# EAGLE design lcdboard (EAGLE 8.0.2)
two capacitors for regulator (in & out) 10uF each
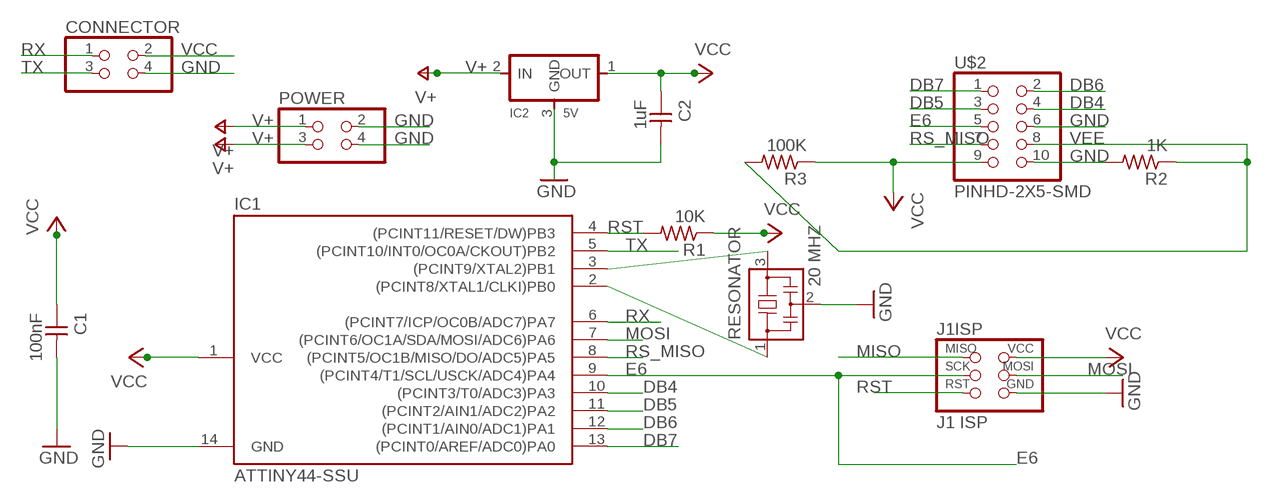
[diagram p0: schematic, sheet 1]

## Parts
C1  100nF  CAP-UNPOLARIZEDFAB  [C1206FAB]
C2  1uF  CAP-UNPOLARIZEDFAB  [C1206FAB]
CONNECTOR  PINHD-2X2-SMD  [2X02SMD]
IC1  ATTINY44-SSU  [SOIC14]
IC2  5V  REGULATORSOT23  [SOT23]
J1ISP  J1 ISP  AVRISPSMD  [2X03SMD]
POWER  PINHD-2X2-SMD  [2X02SMD]
R1  10K  RES-US1206FAB  [R1206FAB]
R2  1K  RES-US1206FAB  [R1206FAB]
R3  100K  RES-US1206FAB  [R1206FAB]
RESONATOR  20 MHZ  RESONATOR  [EFOBM]
U$2  PINHD-2X5-SMD  [2X05SMD]

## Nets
DB4: IC1.10((PCINT3/T0/ADC3)PA3) U$2.4
DB5: IC1.11((PCINT2/AIN1/ADC2)PA2) U$2.3
DB6: IC1.12((PCINT1/AIN0/ADC1)PA1) U$2.2
DB7: IC1.13((PCINT0/AREF/ADC0)PA0) U$2.1
E6: IC1.9((PCINT4/T1/SCL/USCK/ADC4)PA4) J1ISP.3(SCK) U$2.5
GND: C1.2 C2.2 CONNECTOR.4 IC1.14(GND) IC2.3(GND) J1ISP.6(GND) POWER.2 POWER.4 R2.2 RESONATOR.2 U$2.6 U$2.10
MISO: J1ISP.1(MISO)
MOSI: IC1.7((PCINT6/OC1A/SDA/MOSI/ADC6)PA6) J1ISP.4(MOSI)
N$2: IC1.2((PCINT8/XTAL1/CLKI)PB0) RESONATOR.1
N$3: IC1.3((PCINT9/XTAL2)PB1) RESONATOR.3
RS_MISO: IC1.8((PCINT5/OC1B/MISO/DO/ADC5)PA5) U$2.7
RST: IC1.4((PCINT11/RESET/DW)PB3) J1ISP.5(RST) R1.2
RX: CONNECTOR.1 IC1.6((PCINT7/ICP/OC0B/ADC7)PA7)
TX: CONNECTOR.3 IC1.5((PCINT10/INT0/OC0A/CKOUT)PB2)
V+: IC2.2(IN) POWER.1 POWER.3
VCC: C1.1 C2.1 CONNECTOR.2 IC1.1(VCC) IC2.1(OUT) J1ISP.2(VCC) R1.1 R3.1 U$2.9
VEE: R2.1 R3.2 U$2.8

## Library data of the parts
C1 C2 = fab:CAP-UNPOLARIZED
CONNECTOR POWER = fab:PINHD-2X2-SMD
IC1 = fab:ATTINY44
IC2 = fab:REGULATOR
J1ISP = fab:AVRISP
R1-R3 = fab:RES-US: Resistor (US Symbol)
RESONATOR = fab:RESONATOR
U$2 = fab:PINHD-2X5-SMD

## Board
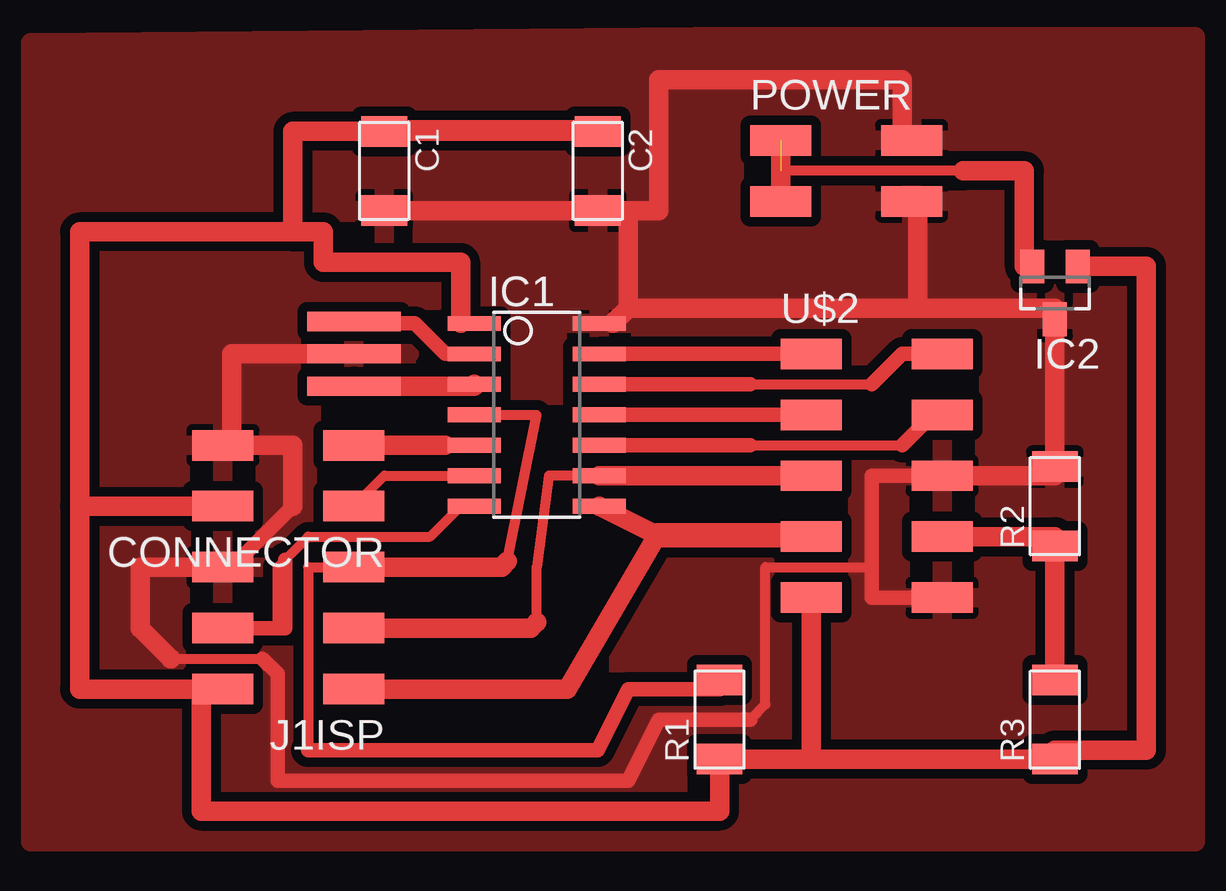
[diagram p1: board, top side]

No outline drawn. Coordinates in mm, seen from the top.
Copper layers (1*16): Top 0.035mm / dielectric 1.5mm / Bottom 0.035mm
Design rules "default *": minimum track width 16mil, minimum drill 24mil, track to track 16mil, track to pad 16mil, pad to pad 16mil, via to via 16mil, smd to smd 8mil, copper to edge 40mil, drill to drill 8mil, minimum pad ring 10mil, minimum via ring 8mil, stop-mask expansion 4mil, vias tented up to drill 0mil, thermal gap 10mil

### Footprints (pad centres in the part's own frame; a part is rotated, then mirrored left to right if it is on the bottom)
C1206FAB = smd 1.27 x 1.905: 1 -1.651,0; 2 1.651,0
2X02SMD = smd 2.54 x 1.27: 1 -2.54,1.27; 2 2.92,1.27; 3 -2.54,-1.27; 4 2.92,-1.27
SOIC14 = smd 0.61 x 2.21: 1 -3.81,-2.603; 2 -2.54,-2.603; 3 -1.27,-2.603; 4 0,-2.603; 5 1.27,-2.603; 6 2.54,-2.603; 7 3.81,-2.603; 8 3.81,2.603; 9 2.54,2.603; 10 1.27,2.603; 11 0,2.603; 12 -1.27,2.603; 13 -2.54,2.603; 14 -3.81,2.603
SOT23 = smd 1 x 1.4: 1 -0.95,-1.1; 2 0.95,-1.1; 3 0,1.1
2X03SMD = smd 2.54 x 1.27: 1 -2.54,2.54; 2 2.92,2.54; 3 -2.54,0; 4 2.92,0; 5 -2.54,-2.54; 6 2.92,-2.54
R1206FAB = smd 1.27 x 1.905: 1 -1.651,0; 2 1.651,0
EFOBM = smd 0.8 x 3.9: 1 -1.35,0; 2 0,0; 3 1.35,0
2X05SMD = smd 2.54 x 1.27: 1 -2.54,2.54; 2 2.92,2.54; 3 -2.54,0; 4 2.92,0; 5 -2.54,-2.54; 6 2.92,-2.54; 7 -2.54,-5.08; 8 2.92,-5.08; 9 -2.54,-7.62; 10 2.92,-7.62

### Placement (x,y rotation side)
C1  13.97,30.48 270 top
C2  22.86,30.48 270 top
CONNECTOR  10.16,17.78 180 top
IC1  20.32,20.32 270 top
IC2  41.91,25.4 180 top
J1ISP  10.16,11.43 180 top
POWER  33.02,30.48 0 top
R1  27.94,7.62 90 top
R2  41.91,16.51 90 top
R3  41.91,7.62 90 top
RESONATOR  12.7,22.86 270 top
U$2  34.29,20.32 0 top

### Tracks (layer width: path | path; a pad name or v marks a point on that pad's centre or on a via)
DB4
  Top 0.406: 29.21,19.05 35.56,19.05 | 36.83,20.32 U$2.4
  Top 0.61: 36.83,20.32 35.56,19.05 | IC1.10 29.21,19.05
DB5
  Top 0.61: U$2.3 IC1.11
DB6
  Top 0.406: U$2.2 36.83,22.86 | 29.21,21.59 34.29,21.59
  Top 0.61: IC1.12 29.21,21.59 | 34.29,21.59 35.56,22.86 U$2.2
DB7
  Top 0.61: U$2.1 IC1.13
E6
  Top 0.406: IC1.9 20.83,17.78 20.32,13.97 20.32,11.68 20.32,11.43 J1ISP.3
  Top 0.813: U$2.5 IC1.9 | J1ISP.3 20.07,11.43 20.32,11.68
GND
  Top 0.406: 13.97,28.57 C1.2 | 35.56,33.02 35.56,31.75 POWER.2 | 10.79,22.86 RESONATOR.2 | 34.92,17.78 U$2.6 | 36.83,12.7 U$2.10 | 36.2,29.21 POWER.4 | 41.91,24.77 IC2.3 R2.2 41.91,17.78 | 9.53,9.53 9.53,6.35 | 29.21,7.62 29.84,8.26 29.84,13.97 34.29,13.97 | 6.99,13.97 J1ISP.6 7.62,13.97 | 5.08,10.16 8.89,10.16
  Top 0.61: U$2.6 34.29,17.78 34.29,13.97 34.29,12.7 38.1,12.7 | 29.21,7.62 25.4,7.62 24.13,5.08 9.53,5.08 9.53,9.53 8.89,10.16 | 10.16,16.51 7.62,13.97
  Top 0.813: 36.2,24.77 36.2,29.21 | 41.91,24.77 36.2,24.77 | 24.13,24.77 23.5,24.13 | 36.2,24.77 24.13,24.77 | IC2.3 41.91,17.78 U$2.6 | C2.2 25.4,28.83 25.4,34.29 35.56,34.29 35.56,31.75 | 10.79,22.86 7.62,22.86 7.62,19.05 CONNECTOR.4 10.16,19.05 10.16,16.51 | C1.2 24.13,28.83 24.13,24.77 | J1ISP.6 3.81,13.97 3.81,11.43 5.08,10.16
  pour Top: 26.92,36.07 47.75,36.07 47.75,2.54 -0.76,2.54 -0.76,35.81
MOSI
  Top 0.406: J1ISP.4 9.53,11.43 9.53,13.97 9.84,14.29 10.79,15.24 15.88,15.24 17.14,16.51 IC1.7
  Top 0.61: J1ISP.4 9.84,11.43 9.84,14.29
N$2
  Top 0.406: 16.51,22.86 IC1.2 | 12.7,24.13 RESONATOR.1
  Top 0.61: 16.51,22.86 15.24,24.13 12.7,24.13
N$3
  Top 0.406: 12.7,21.59 RESONATOR.3
  Top 0.813: RESONATOR.3 17.72,21.51 IC1.3
RS_MISO
  Top 0.813: IC1.8 25.34,15.3 21.59,8.89 13.97,8.89
  Top 1.016: 25.34,15.3 31.75,15.3 U$2.7
RST
  Top 0.406: 22.23,6.35 10.79,6.35 10.79,13.97 J1ISP.5 19.05,13.97 19.1,14.21 20.32,20.32 IC1.4
  Top 0.61: 10.79,6.35 22.86,6.35 24.13,8.89 27.94,8.89 R1.2
  Top 0.813: J1ISP.5 18.86,13.97 19.1,14.21
RX
  Top 0.406: IC1.6 13.97,17.78 CONNECTOR.1
TX
  Top 0.406: 16.51,19.05 IC1.5
  Top 0.813: CONNECTOR.3 16.51,19.05
V+  (1 unrouted)
  Top 0.406: 30.48,30.48 38.1,30.48 40.64,30.48 40.64,26.67 IC2.2
  Top 0.61: POWER.3 POWER.1
  Top 0.813: POWER.1 POWER.3 | IC2.2 40.64,26.5 40.64,30.48 38.1,30.48
VCC
  Top 0.406: 41.91,6.35 43.81,6.35 | 27.94,5.71 R1.1 | 13.97,32.38 22.86,32.38 C2.1 | 17.14,24.13 IC1.1 | CONNECTOR.2 6.99,16.51
  Top 0.813: 31.75,5.97 R1.1 27.94,3.81 6.35,3.81 6.35,8.89 J1ISP.2 1.27,8.89 1.27,16.51 | 31.75,5.97 R3.1 41.91,6.35 45.72,6.35 45.72,26.5 IC2.1 | U$2.9 31.75,5.97 | C2.1 C1.1 10.16,32.13 10.16,27.94 | 1.27,16.51 CONNECTOR.2 | 10.16,27.94 11.43,27.94 11.43,26.67 17.14,26.67 17.14,24.13 | 10.16,27.94 1.27,27.94 1.27,16.51
VEE
  Top 0.406: R3.2 R2.1 41.91,15.24 U$2.8
  Top 0.813: R2.1 R3.2 | U$2.8 41.91,15.24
